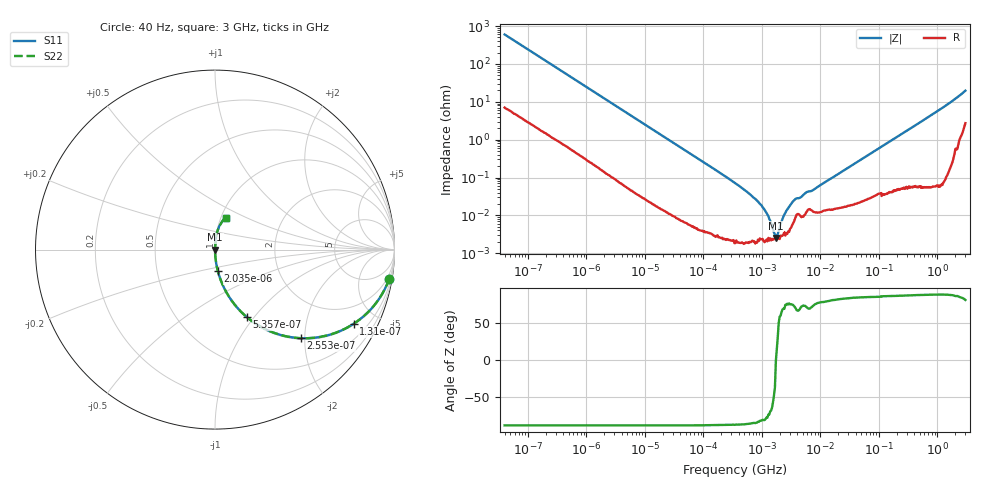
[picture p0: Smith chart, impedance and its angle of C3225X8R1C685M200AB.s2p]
! S-parameter Generated by TDK Corporation
! Copyright(C) 2015 TDK Corporation.
! All Rights Reserved.
! TDK P/N: C3225X8R1C685M200AB (Multilayer Ceramic Chip Capacitors)
! Property: C=6.8uF
! Size(LxWxT): 3.2x2.5x2mm, 0.126x0.098x0.079inches
! Model Type: s2p (Touchstone File Format Version 1.0)
! Frequency: DC=Yes Start=0.00004MHz Stop=3000MHz 568points Log-sweep
! Note: This model was converted from impedance.
! Model Generated on Jun. 23, 2015
! Hash(MD5):
! Port Assignments:
!  1 ---| |--- 2
! Applicable Conditions:
!  Temperature = 25 degC
!  DC Bias Voltage = 0 V
!  Small Signal Operation
! Terms and conditions regarding TDK Simulation Models
! (1)This simulation model is being provided solely for informational purposes. Please refer to the specifications of the products in terms of detailed characteristics of such products.
! (2)In no event shall TDK Corporation of any of its subsidiaries be liable for any loss or damage arising, directly or indirectly,
!  From any information contained in this simulation model, including, but not limited to loss or damages arising from any inaccuracies, omissions or errors in connection with such information.
! (3)Any and all copyrights on this simulation model are owned by TDK Corporation.
!  Duplication or redistribution of this simulation model without prior written permission from TDK Corporation is prohibited.
! (4)This simulation model is subject to any modification or change without any prior notice.
! (5)Neither TDK Corporation nor any of its subsidiaries shall make any warranty, express or implied,
!  Including but not limited to the correctness, implied warranties of merchantability and fitness for a particular purpose with respect to this simulation models.
! (6)The use of this simulation model shall be deemed to have consented to the terms and conditions hereof.
# MHz S MA R 50
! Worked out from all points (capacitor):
!   567 points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, 40 Hz to 3 GHz, reference 50 ohm
!   read as one part in series: C = 6.61 uF near 43.08 Hz
!   lowest |Z| = 2.54 mohm at 1.731 MHz (marker M1)
!   series resonance near 1.735 MHz, so ESL is about 1.3 nH
!   S11 on the Smith chart (normalised r, x): 40 Hz: 1, -12; 131 Hz: 1.04, -3.71; 255.3 Hz: 1.02, -1.91; 535.7 Hz: 1.01, -0.92; 2.035 kHz: 1.00, -0.25; 3 GHz: 1.05, +0.39
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4e-05  0.9845 -9.4  0.1641 79.9  0.1641 79.9  0.9845 -9.4
7.7952e-05  0.9485 -17.8  0.3056 71.5  0.3056 71.5  0.9485 -17.8
0.00013098  0.8759 -28.2  0.4721 61.1  0.4721 61.1  0.8759 -28.2
0.000189754  0.7845 -37.7  0.6109 51.7  0.6109 51.7  0.7845 -37.7
0.000255256  0.6873 -45.9  0.7183 43.4  0.7183 43.4  0.6873 -45.9
0.000535727  0.4152 -64.8  0.9047 24.5  0.9047 24.5  0.4152 -64.8
0.00083584  0.2824 -72.9  0.9559 16.4  0.9559 16.4  0.2824 -72.9
0.002034619  0.1215 -82.4  0.9912 7.0  0.9912 7.0  0.1215 -82.4
0.004952712  0.05074 -86.5  0.9982 2.9  0.9982 2.9  0.05074 -86.5
0.01746572  0.01455 -88.6  0.9997 0.8  0.9997 0.8  0.01455 -88.6
0.3516829  0.0007059 -88.4  1 0.0  1 0.0  0.0007059 -88.4
0.7949038  0.0002613 -85.7  1 0.0  1 0.0  0.0002613 -85.7
1.287042  9.56e-05 -74.5  1 0.0  1 0.0  9.56e-05 -74.5
1.731329  2.538e-05 -0.9  1 0.0  1 0.0  2.538e-05 -0.9
2.328982  9.319e-05 70.2  1 -0.0  1 -0.0  9.319e-05 70.2
3.633676  0.0002617 72.6  0.9999 -0.0  0.9999 -0.0  0.0002617 72.6
4.538749  0.0002968 71.0  0.9999 -0.0  0.9999 -0.0  0.0002968 71.0
5.883347  0.0004157 72.0  0.9999 -0.0  0.9999 -0.0  0.0004157 72.0
7.348767  0.0004574 73.5  0.9999 -0.0  0.9999 -0.0  0.0004574 73.5
149.005  0.008694 86.8  0.9996 -0.5  0.9996 -0.5  0.008694 86.8
997.7393  0.05646 86.1  0.9978 -3.2  0.9978 -3.2  0.05646 86.1
3000  0.1884 71.3  0.9563 -10.8  0.9563 -10.8  0.1884 71.3
